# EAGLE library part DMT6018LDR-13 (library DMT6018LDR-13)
Mosfet Array 60V 8.8A (Ta) 1.9W Surface Mount V-DFN3030-8 Source: Datasheet
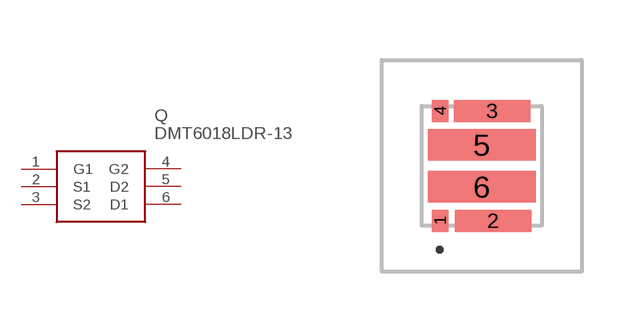
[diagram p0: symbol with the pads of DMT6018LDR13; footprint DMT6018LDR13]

Designator prefix Q

## DMT6018LDR-13 (Arrow_Part_Number: DMT6018LDR-13; Arrow_Price-Stock: https://www.arrow.com/en/products/dmt6018ldr-13/diodes-incorporated?utm_currency=USD&region=nac; Description: Mosfet Array 60V 8.8A (Ta) 1.9W Surface Mount V-DFN3030-8; Height: 0.9mm; Manufacturer_Name: Diodes Incorporated; Manufacturer_Part_Number: DMT6018LDR-13; Mouser_Part_Number: 621-DMT6018LDR-13; Mouser_Price-Stock: https://www.mouser.co.uk/ProductDetail/Diodes-Incorporated/DMT6018LDR-13?qs=1mbolxNpo8cs6AIjMR3%2FiQ%3D%3D)  [DMT6018LDR13]
1  G1
2  S1
3  S2
4  G2
5  D2
6  D1

## Footprint DMT6018LDR13 (pad centres in mm)
DMT6018LDR-13
smd 0.42 x 0.55: 1 -1.037,-1.375; 4 -1.037,1.375
smd 1.92 x 0.55: 2 0.288,-1.375; 3 0.263,1.375
smd 2.7 x 0.79: 5 0,0.525; 6 0,-0.525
